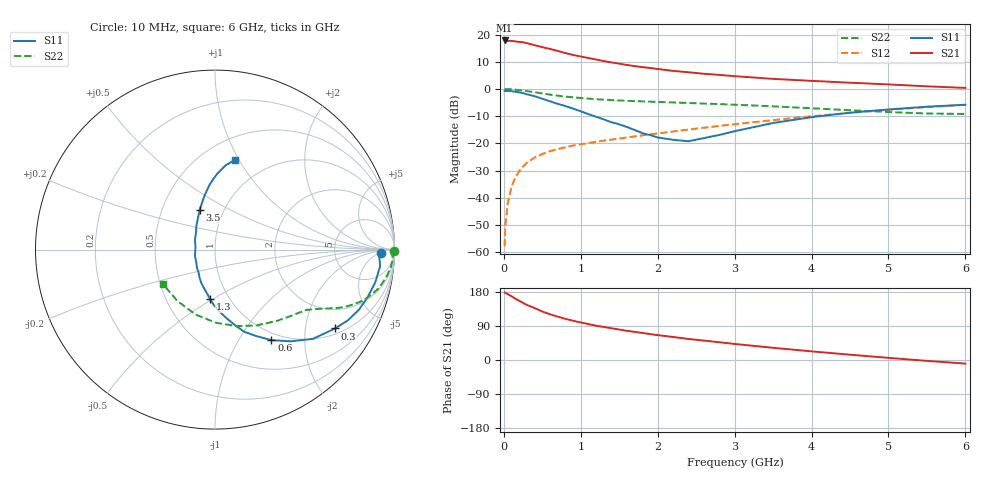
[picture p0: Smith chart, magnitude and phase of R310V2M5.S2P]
! SIEMENS Small Signal Semiconductors
! BFR181
! Si NPN RF Bipolar Junction Transistor in SOT23
! VCE = 10 V  IC = 2.5 mA
! Common Emitter S-Parameters:  May  1996
# GHz  S  MA  R  50
!  f  S11  S21  S12  S22
! GHz  MAG  ANG  MAG  ANG  MAG  ANG  MAG  ANG
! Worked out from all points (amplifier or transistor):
!   36 points, 10 MHz to 6 GHz, reference 50 ohm
!   highest |S21| = 17.8 dB at 10 MHz (marker M1)
!   |S21| within 3 dB of that: start of sweep to 582.7 MHz
!   unconditionally stable (mu >= 1): 1.56 GHz to 3.43 GHz
!   at 250 MHz: K = 0.27, MSG = 22.8 dB, |S12| = -28.4 dB
!   at 1.4 GHz: K = 0.96, MSG = 14.2 dB, |S12| = -18.6 dB
!   at 6 GHz: K = 0.86, MSG = 3.1 dB, |S12| = -5.8 dB
!   S11 on the Smith chart (normalised r, x): 10 MHz: 24, -6; 300 MHz: 1.19, -2.90; 600 MHz: 0.89, -1.39; 1.3 GHz: 0.82, -0.49; 3.5 GHz: 0.77, +0.36; 6 GHz: 0.71, +0.97
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0.01  0.9242 -1.2  7.785 178.3  0.0013 92.7  0.9951 -0.6
0.02  0.9162 -2.3  7.709 177.1  0.0031 89.9  0.9855 -1.2
0.05  0.9247 -5.8  7.649 173.9  0.0079 87.4  0.9921 -2.8
0.1  0.911 -11.7  7.659 168.3  0.016 82.3  0.9847 -5.6
0.15  0.891 -17.1  7.478 161.7  0.024 79.0  0.97 -8.5
0.25  0.8376 -28.2  7.224 150.6  0.0379 73.3  0.9366 -13.3
0.3  0.8003 -33.3  6.954 145.3  0.0444 71.4  0.9139 -15.5
0.4  0.7378 -42.4  6.375 137.0  0.0551 66.7  0.8729 -19.0
0.5  0.6624 -50.5  5.86 127.9  0.0642 63.4  0.8291 -21.6
0.6  0.594 -58.1  5.441 120.7  0.0721 60.8  0.7888 -23.9
0.8  0.4861 -70.4  4.576 108.6  0.0852 57.8  0.7249 -26.8
0.9  0.4379 -74.9  4.219 103.6  0.0916 56.9  0.7038 -27.8
1.1  0.3456 -86.0  3.706 94.8  0.1018 56.5  0.6653 -29.8
1.3  0.2763 -95.7  3.259 87.2  0.1128 56.4  0.6365 -31.4
1.6  0.2002 -112.7  2.76 77.1  0.1288 56.8  0.6064 -33.8
1.9  0.1426 -134.9  2.432 68.5  0.1465 57.1  0.5856 -36.9
2.2  0.1168 -163.1  2.151 60.7  0.166 57.2  0.5665 -40.2
2.4  0.1098 172.5  2.029 55.6  0.1796 57.1  0.5538 -42.7
3.5  0.2377 111.1  1.534 32.2  0.2679 52.7  0.4807 -61.6
4.5  0.3676 94.3  1.305 14.0  0.3645 44.3  0.4074 -89.4
5.5  0.4729 82.9  1.12 -2.3  0.465 32.5  0.3546 -126.2
6  0.5139 77.2  1.047 -9.5  0.5116 25.6  0.3478 -146.6
